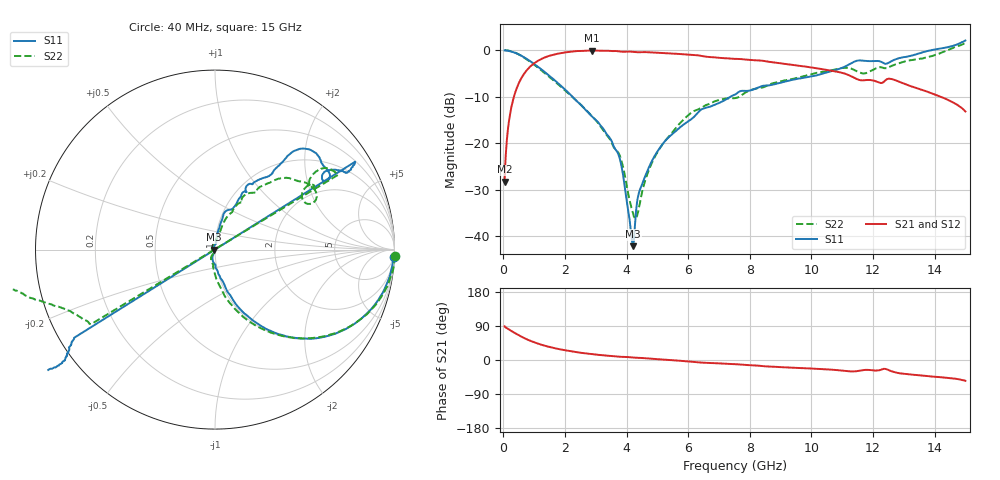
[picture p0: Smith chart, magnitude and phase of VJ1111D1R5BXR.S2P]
! VJ1111D1R5BXR
! DATE 03/08/2022  10:38
! CAPACITORS MOUNTED IN SERIES ON 25 MIL THICK MICROSTRIP SUBSTRATE
# GHz  S  MA  R  50.00
!  FREQ  S11M  S11A  S21M  S21A  S12M  S12A  S22M  S22A
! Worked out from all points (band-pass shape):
!   801 points, 40 MHz to 15 GHz, reference 50 ohm
!   highest |S21| = -0.07 dB at 2.864 GHz (marker M1); lowest = -28.2 dB at 40 MHz (marker M2)
!   |S21| within 3 dB of the highest: 948.1 MHz to 9.316 GHz (8.368 GHz wide, 163 % of centre)
!   lowest |S11| = -42.1 dB at 4.21 GHz (marker M3), VSWR 1.02, Z = 49.2 - j0.0291 ohm
!   |S11| at or under -10 dB: 2.242 GHz to 7.364 GHz (5.123 GHz wide, 107 % of centre)
!   |S22| runs from -36.2 to 1.6 dB; largest |S21 - S12| = 0.006
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0.04  0.9968 -2.2  0.03875 89.0  0.03887 87.0  1.005 -2.1
0.1522  0.986 -8.0  0.1456 82.0  0.1455 82.1  0.9929 -8.1
0.2644  0.967 -13.9  0.2484 76.3  0.2483 76.2  0.9729 -13.9
0.6571  0.8445 -32.1  0.5486 58.6  0.5485 58.6  0.8416 -32.1
1.5173  0.5238 -57.3  0.8768 33.9  0.8727 34.0  0.5092 -59.6
2.5458  0.2547 -72.8  0.9819 18.7  0.9797 18.8  0.252 -78.9
2.8637  0.1962 -75.3  0.9921 15.6  0.9901 15.6  0.1985 -83.2
3.7426  0.07486 -95.0  0.9728 8.7  0.9707 8.8  0.07815 -101.4
4.2101  0.007837 -177.8  0.9602 6.4  0.9586 6.5  0.01777 -123.2
4.3223  0.02083 105.2  0.9513 6.0  0.9498 6.1  0.01602 -162.2
4.4345  0.03187 82.2  0.9542 5.8  0.9524 5.9  0.0227 132.5
4.6776  0.05065 81.1  0.9524 4.2  0.95 4.3  0.04713 89.0
5.0329  0.08445 81.6  0.9384 2.0  0.936 2.2  0.08284 77.1
6.0988  0.1813 76.7  0.8919 -4.3  0.8903 -4.2  0.2128 67.9
7.52  0.3339 64.1  0.8071 -11.0  0.8056 -10.8  0.3057 60.4
10.0258  0.5256 53.2  0.6509 -22.6  0.6481 -22.4  0.5549 46.1
11.3722  0.7487 48.8  0.5088 -30.2  0.5078 -30.0  0.6177 25.8
12.5129  0.7352 35.1  0.4946 -26.8  0.4935 -26.6  0.655 36.5
13.4105  0.9066 31.3  0.3922 -39.6  0.3915 -39.3  0.7975 32.6
13.5788  0.943 -147.3  0.3758 -40.9  0.3739 -40.5  0.813 -150.1
14.5138  1.093 -143.6  0.2835 -47.8  0.2834 -47.5  1.032 -164.2
15  1.274 -147.6  0.2196 -54.9  0.2193 -54.3  1.198 -170.6
